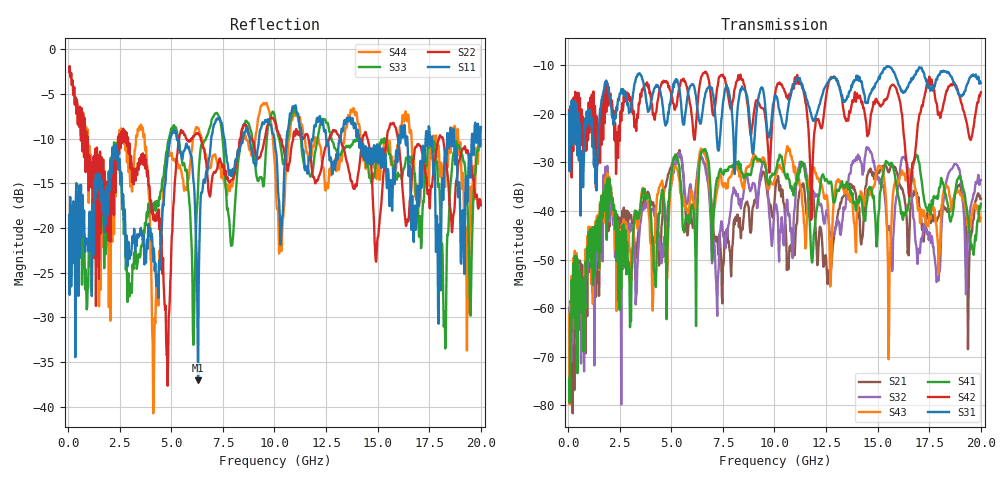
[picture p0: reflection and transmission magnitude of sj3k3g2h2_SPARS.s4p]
! FILE: E:\users\goganessyan\GBX_Backplane\FR408_backplane\1m_INBOUND_NEXT\sj3k3g2h2_SPARS.s4p
# MHZ S RI R 50.00
! FREQ  S11  S12  S13  S14
!  S21  S22  S23  S24
!  S31  S32  S33  S34
!  S41  S42  S43  S44
!  REAL  IMAG  REAL  IMAG  REAL  IMAG  REAL  IMAG
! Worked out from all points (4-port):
!   799 points, 50 MHz to 20 GHz, reference 50 ohm
!   strongest paths, dB at 50 MHz, 5.025 GHz, 10.03 GHz, 15.03 GHz, 20 GHz:
!     S31: -19.7, -15.7, -16.2, -13.0, -13.6
!     S42: -19.2, -16.3, -16.0, -17.6, -15.5
!     S41: -74.8, -31.5, -32.2, -41.4, -38.5
!     S43: -61.1, -33.4, -33.2, -30.7, -41.5
!     S32: -59.9, -33.8, -39.1, -33.5, -33.6
!     S21: -64.2, -30.4, -36.6, -31.9, -37.5
!   lowest |S11| = -37.0 dB at 6.3 GHz (marker M1), VSWR 1.03, Z = 48.8 - j0.615 ohm
!   |S11| at or under -10 dB: start of sweep to 4.948 GHz; 5.271 GHz to 6.937 GHz (1.666 GHz wide, 27.3 % of centre); 14.09 GHz to 16.01 GHz (1.925 GHz wide, 12.8 % of centre)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
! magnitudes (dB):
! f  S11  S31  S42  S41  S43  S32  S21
! 50 MHz  -18.6  -19.7  -19.2  -74.8  -61.1  -59.9  -64.2
! 1.975 GHz  -13.8  -15.6  -14.5  -35.4  -33.9  -32.9  -33.7
! 3.6 GHz  -20.8  -12.9  -14.9  -36.4  -35.5  -39.6  -38.3
! 4.15 GHz  -22.2  -15.2  -20.0  -52.0  -48.3  -39.8  -39.2
! 6.3 GHz  -37.0  -20.1  -16.7  -35.4  -31.5  -30.7  -31.7
! 7.225 GHz  -7.8  -26.0  -14.6  -33.2  -35.6  -61.6  -45.4
! 20 GHz  -8.7  -13.6  -15.5  -38.5  -41.5  -33.6  -37.5
